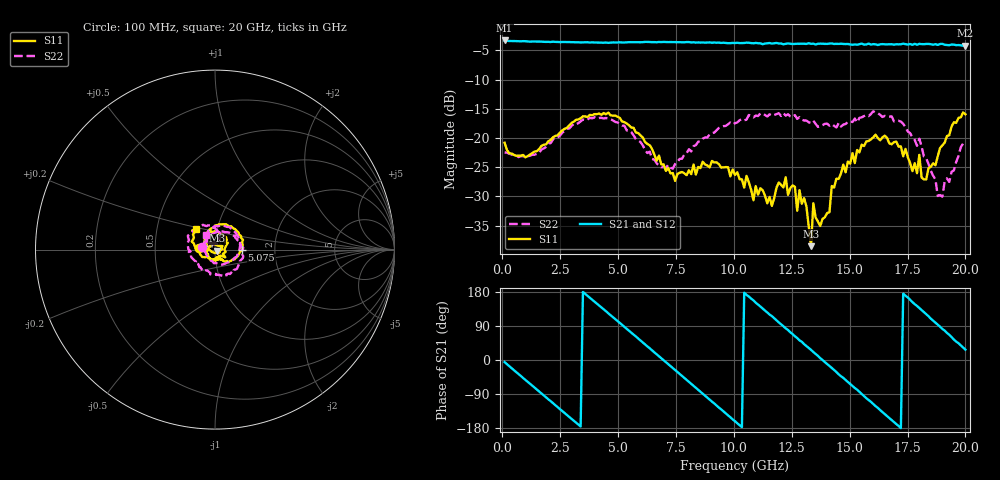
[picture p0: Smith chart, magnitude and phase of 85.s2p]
!Agilent Technologies,N5230C,MY49001569,A.09.33.09
!Agilent N5230C: A.09.33.09
!Date: Tuesday, July 28, 2015 17:44:39
!Correction: S11(Full 2 Port(1,2))
!S21(Full 2 Port(1,2))
!S12(Full 2 Port(1,2))
!S22(Full 2 Port(1,2))
!S2P File: Measurements: S11, S21, S12, S22:
# Hz S  dB  R 50
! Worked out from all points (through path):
!   201 points, 100 MHz to 20 GHz, reference 50 ohm
!   highest |S21| = -3.28 dB at 100 MHz (marker M1); lowest = -4.2 dB at 20 GHz (marker M2)
!   group delay of S21, straight-line fit = 146 ps
!   lowest |S11| = -38.5 dB at 13.33 GHz (marker M3), VSWR 1.02, Z = 51.1 - j0.564 ohm
!   |S11| at or under -10 dB: start of sweep to end of sweep
!   |S22| runs from -30.0 to -15.4 dB; largest |S21 - S12| = 0.017
!   S11 on the Smith chart (normalised r, x): 100 MHz: 0.83, +0.02; 5.075 GHz: 1.35, -0.01; 20 GHz: 0.78, +0.19
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1e8  -20.81 173.6  -3.28 -5.6  -3.25 -6.2  -22.45 169.7
1.7915e9  -21.16 130.2  -3.49 -93.4  -3.49 -93.5  -21.78 136.2
3.483e9  -16.28 67.0  -3.62 179.5  -3.61 179.8  -16.82 71.7
5.075e9  -16.55 -1.2  -3.60 97.8  -3.60 97.8  -17.57 -8.4
6.7665e9  -23.02 -54.6  -3.54 10.0  -3.56 9.9  -24.72 -133.3
7.463e9  -27.35 -58.0  -3.56 -26.7  -3.58 -26.7  -24.45 159.8
8.458e9  -24.96 -79.2  -3.62 -78.5  -3.59 -78.5  -20.64 93.0
1.005e10  -26.32 -153.0  -3.73 -161.4  -3.68 -161.7  -17.45 25.8
1.0846e10  -30.66 145.9  -3.77 157.4  -3.77 156.9  -16.47 -1.7
1.1841e10  -28.52 45.1  -3.71 104.8  -3.79 104.6  -15.91 -38.1
1.2637e10  -28.34 2.7  -3.87 62.6  -3.84 62.8  -16.08 -65.8
1.27365e10  -32.46 -29.4  -3.85 58.0  -3.84 57.5  -16.71 -70.7
1.2836e10  -28.93 1.5  -3.85 51.9  -3.79 52.6  -16.43 -73.9
1.33335e10  -38.53 -27.8  -3.87 26.8  -3.94 25.6  -17.39 -99.3
1.3433e10  -31.18 -52.4  -3.83 21.1  -3.91 20.7  -17.04 -100.9
1.37315e10  -35.08 -109.8  -3.83 4.8  -3.88 5.2  -17.97 -114.3
1.53235e10  -22.05 134.2  -4.02 -78.3  -3.80 -79.0  -17.30 -175.8
1.67165e10  -20.92 73.8  -3.94 -153.4  -3.97 -153.9  -16.34 119.6
1.7612e10  -24.28 15.5  -3.89 158.8  -4.00 158.6  -19.14 84.7
1.85075e10  -24.91 -108.1  -3.93 109.0  -3.93 110.4  -25.62 69.8
1.9005e10  -21.27 -161.8  -3.86 82.0  -3.92 82.1  -30.04 118.7
2e10  -15.94 132.8  -4.20 27.4  -4.24 26.8  -20.52 122.1
